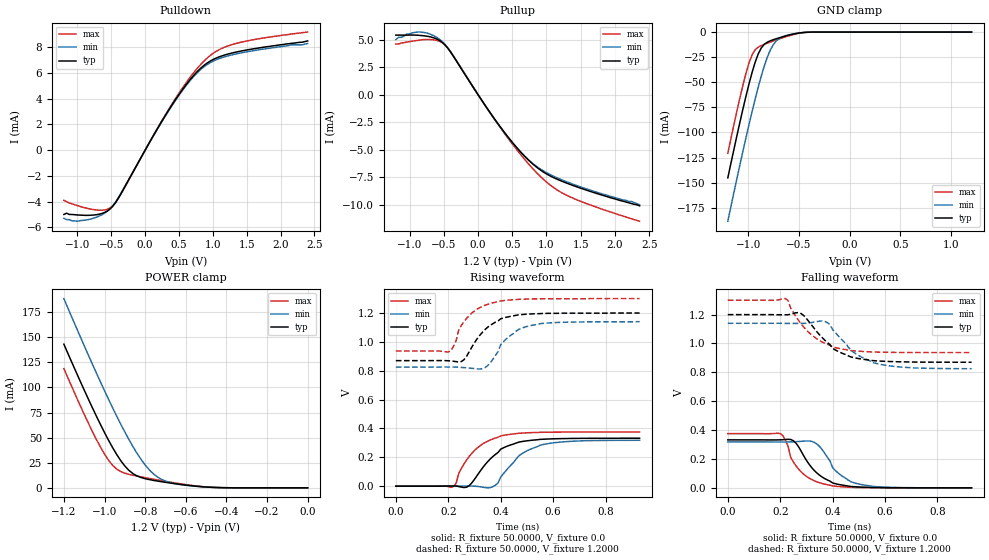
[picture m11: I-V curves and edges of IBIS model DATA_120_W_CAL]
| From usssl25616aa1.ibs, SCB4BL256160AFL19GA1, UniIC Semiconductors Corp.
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|   Model DATA_120_W_CAL
[Model]  DATA_120_W_CAL
Model_type I/O
Polarity   Non-Inverting
Enable   Active-High
Vinl =   0.3800V
Vinh =   0.8200V
Vmeas =  0.6000V
Cref =   5.0000pF
Rref =   50.0000
Vref =   0.6000V
C_comp   1.7430pF   1.7110pF   1.7640pF
[Temperature Range]   25.0000   0.1250k   -40.0000
[Voltage Range]   1.2000V   1.1400V   1.3000V
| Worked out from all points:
|   slope of the pulldown table from 0 to 0.18 V, typ, clamps not added: 108 ohm
|   slope of the pullup table from 0 to 0.18 V, typ, clamps not added: 108 ohm
|   GND clamp passes 1 mA (typ) near -0.50 V on its own axis
|   POWER clamp passes 1 mA (typ) near -0.51 V on its own axis
|   rising waveform, R_fixture 50.0000, V_fixture 0.0: 20-80 % time 103ps typ, 111ps min, 101ps max; typ from 0 V to 0.332 V
|   rising waveform, R_fixture 50.0000, V_fixture 1.2000: 20-80 % time 96ps typ, 87.9ps min, 80.3ps max; typ from 0.87 V to 1.2 V
|   falling waveform, R_fixture 50.0000, V_fixture 0.0: 20-80 % time 91.6ps typ, 87.9ps min, 76.6ps max; typ from 0.332 V to 0 V
|   falling waveform, R_fixture 50.0000, V_fixture 1.2000: 20-80 % time 115ps typ, 122ps min, 116ps max; typ from 1.2 V to 0.87 V
[Pulldown]
|Voltage   I(typ)   I(min)   I(max)
-1.2V     -5mA       -5.3mA     -3.9mA
-1V       -5.04mA    -5.53mA    -4.31mA
-800mV    -5.059mA   -5.35mA    -4.59mA
-600mV    -4.846mA   -4.908mA   -4.649mA
-480mV    -4.371mA   -4.331mA   -4.339mA
-360mV    -3.417mA   -3.37mA    -3.43mA
400mV     3.547mA    3.496mA    3.616mA
680mV     5.593mA    5.511mA    5.776mA
880mV     6.641mA    6.53mA     6.99mA
1.08V     7.232mA    7.098mA    7.783mA
1.32V     7.603mA    7.46mA     8.27mA
2.4V      8.5mA      8.3mA      9.19mA
[Pullup]
|Voltage   I(typ)   I(min)   I(max)
-1.2V     5.4mA      5mA        4.6mA
-1.04V    5.4mA      5.5mA      4.77mA
-840mV    5.37mA     5.68mA     4.96mA
-680mV    5.219mA    5.442mA    4.989mA
-520mV    4.73mA     4.797mA    4.698mA
-400mV    3.86mA     3.889mA    3.883mA
360mV     -3.215mA   -3.252mA   -3.291mA
600mV     -5.052mA   -5.069mA   -5.267mA
800mV     -6.3mA     -6.257mA   -6.722mA
1.04V     -7.336mA   -7.214mA   -8.14mA
1.28V     -8mA       -7.879mA   -9.095mA
2.36V     -10.1mA    -10mA      -11.5mA
[GND_clamp]
|Voltage   I(typ)   I(min)   I(max)
-1.2V     -145.3mA   -188.5mA   -120.8mA
-1.05V    -76.2mA    -118.2mA   -52.43mA
-990mV    -51.2mA    -91.62mA   -30.39mA
-960mV    -39.9mA    -78.82mA   -22.48mA
-900mV    -21.67mA   -54.7mA    -15mA
-870mV    -15.78mA   -43.66mA   -13.45mA
-810mV    -10.04mA   -24.79mA   -11.07mA
-780mV    -8.658mA   -17.59mA   -9.958mA
-720mV    -6.57mA    -8.545mA   -7.793mA
-630mV    -3.906mA   -3.64mA    -4.741mA
-420mV    -215.4uA   -240.5uA   -235uA
1.2V      1.597nA    22.84nA    1.463nA
[POWER_clamp]
|Voltage   I(typ)   I(min)   I(max)
-1.2V     143mA      188.4mA    118.7mA
-1.1V     97.38mA    141.5mA    73.24mA
-1.04V    71.38mA    114.3mA    48.22mA
-1V       55.04mA    96.69mA    33.64mA
-960mV    40mA       79.65mA    22.42mA
-900mV    21.75mA    55.6mA     14.58mA
-860mV    14.17mA    41.05mA    12.52mA
-800mV    9.133mA    22.79mA    10.12mA
-740mV    6.786mA    10.88mA    7.886mA
-660mV    4.332mA    4.436mA    5.101mA
-520mV    1.103mA    1.063mA    1.274mA
0V        1.597nA    6.003nA    2.16nA
[Ramp]
| variable   typ   min   max
dV/dt_r  0.1993/0.1052n   0.1908/0.1129n   0.2253/95.2293p
dV/dt_f  0.1979/0.1159n   0.1887/0.1223n   0.2179/0.1078n
R_load = 50.0000
[Rising Waveform]
R_fixture= 50.0000
V_fixture= 0.0
V_fixture_min= 0.0
V_fixture_max= 0.0
|time   V(typ)   V(min)   V(max)
0s        0V         0V         0V
220ps     1.212mV    173.8uV    -2.406mV
250ps     -6.397mV   774.5uV    122.7mV
290ps     22.9mV     959.1uV    228.1mV
360ps     188.1mV    -10.3mV    320mV
390ps     233.7mV    22.89mV    339.1mV
400ps     256.1mV    63.18mV    348.1mV
470ps     305.5mV    211.6mV    366.7mV
550ps     324.1mV    283.7mV    373mV
930ps     332.2mV    318mV      375.5mV
[Rising Waveform]
R_fixture= 50.0000
V_fixture= 1.2000
V_fixture_min= 1.1400
V_fixture_max= 1.3000
|time   V(typ)   V(min)   V(max)
0s        870mV      825.1mV    936.9mV
200ps     869.1mV    825.5mV    930.2mV
220ps     865.7mV    825.5mV    969mV
250ps     863.8mV    823mV      1.114V
290ps     964.1mV    816.8mV    1.2V
340ps     1.085V     821.4mV    1.254V
400ps     1.16V      980.4mV    1.284V
470ps     1.188V     1.088V     1.295V
550ps     1.196V     1.126V     1.298V
930ps     1.2V       1.14V      1.3V
[Falling Waveform]
R_fixture= 50.0000
V_fixture= 0.0
V_fixture_min= 0.0
V_fixture_max= 0.0
|time   V(typ)   V(min)   V(max)
0s        332.3mV    318.2mV    375.5mV
200ps     332.6mV    317.9mV    376.1mV
220ps     334.6mV    317.8mV    330.4mV
240ps     335.1mV    318.7mV    211.1mV
280ps     253.3mV    322.2mV    110.4mV
330ps     120mV      315.1mV    48.67mV
400ps     33.77mV    139.9mV    13.1mV
470ps     9.429mV    41.79mV    3.526mV
550ps     2.241mV    10.46mV    805uV
930ps     3.658uV    22.09uV    1.051uV
[Falling Waveform]
R_fixture= 50.0000
V_fixture= 1.2000
V_fixture_min= 1.1400
V_fixture_max= 1.3000
|time   V(typ)   V(min)   V(max)
0s        1.2V       1.14V      1.3V
220ps     1.199V     1.139V     1.311V
280ps     1.207V     1.139V     1.135V
320ps     1.127V     1.145V     1.059V
370ps     1.023V     1.153V     1.002V
390ps     991.8mV    1.131V     987.8mV
420ps     945.9mV    1.056V     967.4mV
480ps     902.4mV    938.9mV    949.3mV
570ps     879.4mV    860.3mV    940.3mV
930ps     870.1mV    825.5mV    936.9mV
